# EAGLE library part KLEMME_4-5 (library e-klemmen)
Klemme 4 5
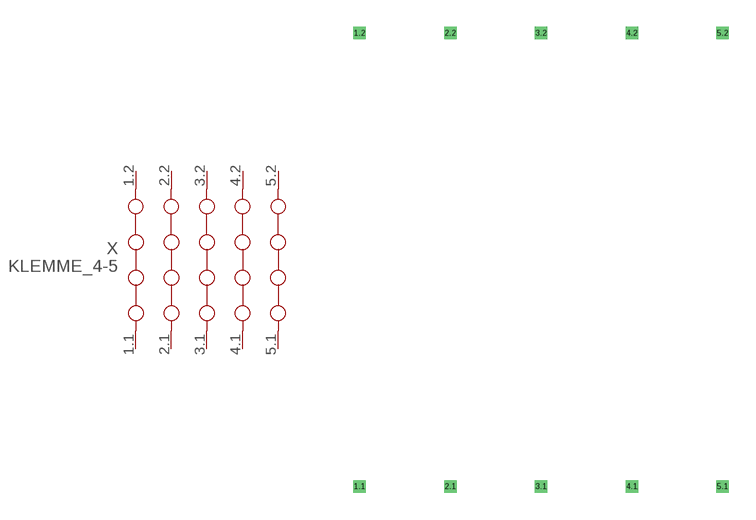
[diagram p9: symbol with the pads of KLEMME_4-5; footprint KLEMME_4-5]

Designator prefix X

## KLEMME_4-5  [KLEMME_4-5]
1.1  1.1  pas
1.2  1.2  pas
2.1  2.1  pas
2.2  2.2  pas
3.1  3.1  pas
3.2  3.2  pas
4.1  4.1  pas
4.2  4.2  pas
5.1  5.1  pas
5.2  5.2  pas

## Footprint KLEMME_4-5 (pad centres in mm)
Dummy
drill 0.2 pad 0.6 square: 1.1 0,-12.7; 1.2 0,12.7; 2.1 5.08,-12.7; 2.2 5.08,12.7; 3.1 10.16,-12.7; 3.2 10.16,12.7; 4.1 15.24,-12.7; 4.2 15.24,12.7; 5.1 20.32,-12.7; 5.2 20.32,12.7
